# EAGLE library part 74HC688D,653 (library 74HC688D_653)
74HC688 - 8-bit magnitude comparator@en-us Source: Datasheet
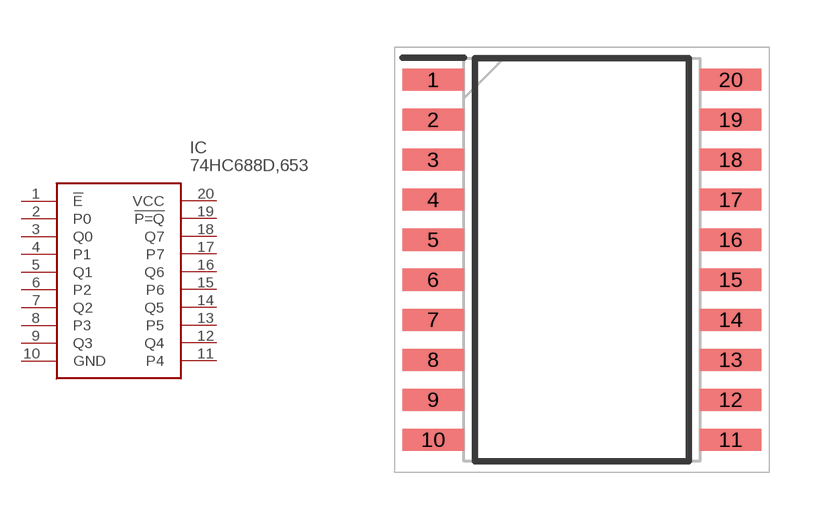
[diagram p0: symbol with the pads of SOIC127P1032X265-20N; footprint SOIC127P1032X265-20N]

Designator prefix IC

## 74HC688D,653 (Description: 74HC688 - 8-bit magnitude comparator@en-us; Height: 2.65mm; Manufacturer_Name: Nexperia; Manufacturer_Part_Number: 74HC688D,653; Mouser_Part_Number: 771-74HC688D-T; Mouser_Price-Stock: https://www.mouser.co.uk/ProductDetail/Nexperia/74HC688D653?qs=P62ublwmbi%252BZYv%2F8J45taw%3D%3D)  [SOIC127P1032X265-20N]
1  !E
2  P0
3  Q0
4  P1
5  Q1
6  P2
7  Q2
8  P3
9  Q3
10  GND
11  P4
12  Q4
13  P5
14  Q5
15  P6
16  Q6
17  P7
18  Q7
19  !P=Q
20  VCC

## Footprint SOIC127P1032X265-20N (pad centres in mm)
SOT163-1
smd 1.95 x 0.7: 1 -4.725,5.715; 2 -4.725,4.445; 3 -4.725,3.175; 4 -4.725,1.905; 5 -4.725,0.635; 6 -4.725,-0.635; 7 -4.725,-1.905; 8 -4.725,-3.175; 9 -4.725,-4.445; 10 -4.725,-5.715; 11 4.725,-5.715; 12 4.725,-4.445; 13 4.725,-3.175; 14 4.725,-1.905; 15 4.725,-0.635; 16 4.725,0.635; 17 4.725,1.905; 18 4.725,3.175; 19 4.725,4.445; 20 4.725,5.715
